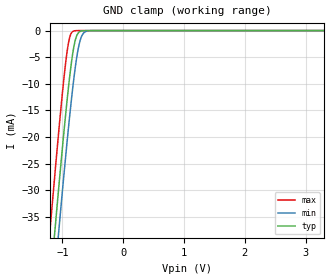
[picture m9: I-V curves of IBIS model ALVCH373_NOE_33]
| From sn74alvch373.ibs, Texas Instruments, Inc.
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[Model]   ALVCH373_NOE_33
Model_type  Input
Vinl=0.8
Vinh=2.0
| variable   typ   min   max
C_comp   3.57pF   2.91pF   4.36pF
[Temperature Range]   40   100   -40
| Ambient temperature   25   85   -40
[Voltage range]   3.3   3   3.6
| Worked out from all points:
|   GND clamp passes 1 mA (typ) near -0.77 V on its own axis
[GND Clamp]
| ALVCH373_NOE_33
|   Voltage   I(typ)   I(min)   I(max)
-3.3V     -341.5mA   -348.9mA   -332.3mA
-1.215V   -49.6mA    -57.88mA   -38.96mA
-1.185V   -45.62mA   -53.91mA   -34.98mA
-1.125V   -37.77mA   -46.06mA   -27.13mA
-1.065V   -30.08mA   -38.33mA   -19.51mA
-920mV    -12.75mA   -20.53mA   -3.718mA
-875mV    -8.124mA   -15.45mA   -1.065mA
-825mV    -3.922mA   -10.26mA   -137.1uA
-775mV    -1.291mA   -5.83mA    -13.57uA
-715mV    -205.4uA   -2.128mA   -808.5nA
-585mV    -2.266uA   -70.82uA   -1.783nA
3.3V      6.304pA    9.258pA    5.93pA
